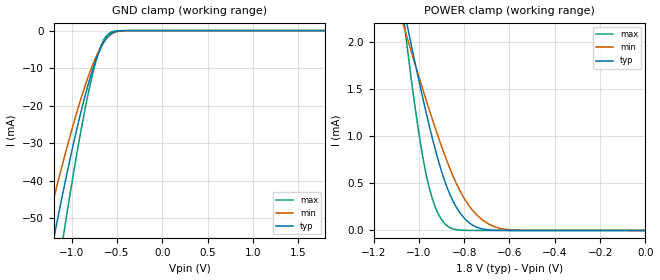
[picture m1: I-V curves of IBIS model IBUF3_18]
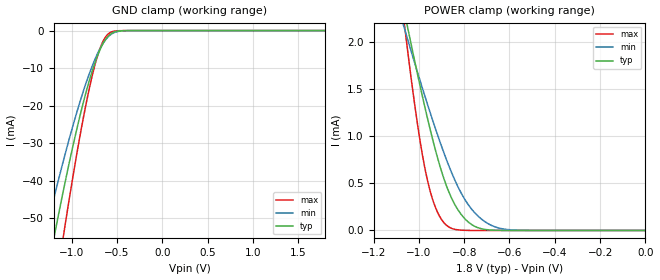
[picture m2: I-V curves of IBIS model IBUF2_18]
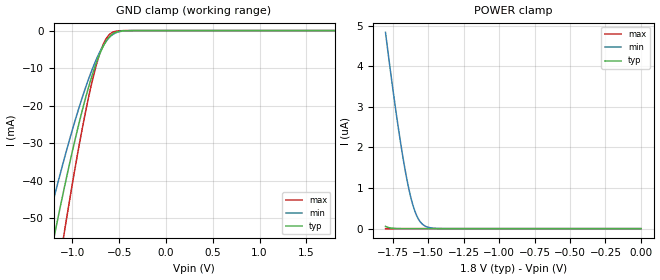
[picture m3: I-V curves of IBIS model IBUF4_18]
| TEXAS INSTRUMENTS INCORPORATED
| High Precision Analog Group
| IBIS Model of TLV320AIC3204
| Ultra Low Power Stereo Audio Codec
| part#   Digital Voltage Range   Package-type   #pin
| TLV320AIC3204RHBT   1.65V-1.95V   QFN   32
| TLV320AIC3204RHBR   1.65V-1.95V   QFN   32
[IBIS Ver]   4.0
[Comment char]  |_char
[File Name]   tlv320aic3204.ibs
[File Rev]   1.2 | E
[Date]   April 10, 2012
[Source]   Data created from TI-SPICE simulations at TI-HPA.
[Notes]   IBIS models created for IOVDD=DVDD=1.8/1.65/1.95 voltage range.
[Disclaimer] Property of Texas Instruments Incorporated.  Unauthorized
   reproduction and/or distribution is strictly prohibited.
   This product is protected under copyright law.
   Created  2012, (C) Copyright  2008, Texas Instruments
   Incorporated, All Rights Reserved
   UNLESS THERE IS A SIGNED, WRITTEN AGREEMENT TO THE
   CONTRARY, TEXAS INSTRUMENTS (TI) IS PROVIDING THE IBIS
   MODELS  AND WITHOUT ANY WARRANTY, EXPRESSED OR
   IMPLIED.  TI assumes no liability for:
   1) the accuracy of the IBIS models provided to your
   company;
   2) the proper functioning of these IBIS Models in your
   design or for any resulting applications; or
   3) infringement of patents, copyrights or intellectual
   property rights resulting from your use of these IBIS
   models.
   TI provides IBIS Models as a service to our customers.
   You and your company shall not distribute, sell or give
   these models to anyone else without prior written
   permission from TI.
   TI reserves the right to make changes to our products or
   to discontinue any semiconductor product or service
   without notice, and advises our customers to obtain the
   latest version of relevant information to verify, before
   placing orders, that the information being relied on is
   current.
   Please be aware that your receipt and use of the IBIS
   information provided shall serve as acceptance of these
   terms and conditions.  If you do not accept these terms,
   you should return or destroy the IBIS models and any
   other accompanying information immediately.
| Component TLV320AIC3204
[Component]   TLV320AIC3204
[Manufacturer]   Texas Instruments, Inc.
[Package]
|   typ   min   max
R_pkg   0.0761   0.0299   0.1101
L_pkg   1.1413nH   0.7391nH   1.5998nH
C_pkg   0.1818pF   0.1548pF   0.2745pF
[Pin]   signal_name   model_name   R_pin   L_pin   C_pin
1   MCLK   IBUF3_18   0.0843   1.21035nH   0.15565pF
2   BCLK   IOBUF_18   0.07376   1.04734nH   0.16399pF
3   WCLK   IOBUF_18   0.06637   0.94061nH   0.15628pF
4   DIN_MFP1   IBUF3_18   0.06804   0.96386nH   0.15867pF
5   DOUT_MFP2   OBUF2_18   0.07842   1.11449nH   0.17348pF
6   IOVDD   POWER   0.09718   1.3981nH   0.1889pF
7   IOVSS   GND   0.07358   1.04468nH   0.16245pF
8   SCLK_MFP3   IBUF4_18   0.08662   1.24526nH   0.15856pF
9   SCL_SSZ   I2CBUF_18   0.09486   1.37075nH   0.16588pF
10   SDA_MOSI   I2CBUF_18   0.08551   1.22071nH   0.17615pF
11   MISO_MFP4   OBUF1_18   0.08354   1.1883nH   0.1739pF
12   SPI_SELECT   IBUF1_18   0.08888   1.26731nH   0.17521pF
13   IN1_L   NC   0.10506   1.52032nH   0.19276pF
14   IN1_R   NC   0.09092   1.30262nH   0.18492pF
15   IN2_L   NC   0.0837   1.19263nH   0.17435pF
16   IN2_R   NC   0.095   1.36986nH   0.17145pF
17   AVSS   GND   0.04502   0.98171nH   0.20452pF
18   REF   NC   0.07598   1.07406nH   0.17015pF
19   MICBIAS   NC   0.08288   1.1762nH   0.17166pF
20   IN3_L   NC   0.07046   0.99184nH   0.16153pF
21   IN3_R   NC   0.06587   0.92585nH   0.15484pF
22   LOL   NC   0.06756   0.95011nH   0.15852pF
23   LOR   NC   0.0803   1.1385nH   0.17871pF
24   AVDD   POWER   0.0437   0.89119nH   0.20777pF
25   HPL   NC   0.11011   1.59985nH   0.18762pF
26   LDOIN_HPVDD   POWER   0.04871   1.0902nH   0.22686pF
27   HPR   NC   0.0491   0.74997nH   0.27451pF
28   DVSS   GND   0.04558   1.00319nH   0.21651pF
29   DVDD   POWER   0.02991   0.73918nH   0.25324pF
30   LDO_SELECT   NC   0.08352   1.18799nH   0.17586pF
31   RESETB   IBUF2_18   0.08629   1.23261nH   0.17795pF
32   GPIO_MFP5   IOBUF_18   0.09629   1.39283nH   0.16735pF
| Models and submodels in the file (8): IBUF3_18 (Input), IBUF1_18 (Input), IBUF2_18 (Input), IBUF4_18 (Input), IOBUF_18 (I/O), I2CBUF_18 (I/O_open_drain), OBUF2_18 (Output), OBUF1_18 (Output)
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[Model]   IBUF3_18
Model_type  Input
Vinl=0.495
Vinh=1.365
| variable   typ   min   max
C_comp   1.31pF   1.15pF   1.43pF
[Temperature Range]   40   100   -40
| Ambient temperature   25   85   -40
[Voltage range]   1.8   1.65   1.95
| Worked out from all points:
|   GND clamp passes 1 mA (typ) near -0.57 V on its own axis
|   POWER clamp passes 1 mA (typ) near -0.94 V on its own axis
[GND Clamp]
| IBUF3_18
|   Voltage   I(typ)   I(min)   I(max)
-1.8V     -137.6mA   -110mA     -176.5mA
-1.29V    -67.21mA   -54.1mA    -87.09mA
-1.18V    -53.33mA   -43.13mA   -68.94mA
-1.08V    -41.34mA   -33.68mA   -53.07mA
-910mV    -22.93mA   -19.14mA   -28.35mA
-785mV    -11.72mA   -10.2mA    -13.28mA
-730mV    -7.711mA   -6.953mA   -8.032mA
-675mV    -4.471mA   -4.268mA   -4.022mA
-625mV    -2.333mA   -2.42mA    -1.689mA
-575mV    -1.009mA   -1.184mA   -542.1uA
-390mV    -10.81uA   -26.47uA   -1.124uA
1.8V      39.03pA    509.5pA    14.13pA
[POWER Clamp]
| IBUF3_18
|   Voltage   I(typ)   I(min)   I(max)
-1.8V     11.83mA    8.628mA    19.35mA
-1.065V   2.333mA    2.152mA    2.209mA
-1.055V   2.216mA    2.07mA     2.012mA
-1.045V   2.1mA      1.989mA    1.819mA
-1V       1.591mA    1.63mA     1.031mA
-960mV    1.169mA    1.323mA    510.8uA
-915mV    749uA      995.8uA    180.4uA
-860mV    365.8uA    639.8uA    27.05uA
-815mV    175.7uA    404.5uA    3.749uA
-775mV    76.29uA    250.6uA    597.6nA
-655mV    1.92uA     31.22uA    2.358nA
-16.28fV  39.03pA    476.1pA    17.07pA
[Model]   IBUF2_18
Model_type  Input
Vinl=0.495
Vinh=1.365
| variable   typ   min   max
C_comp   1.31pF   1.15pF   1.42pF
[Temperature Range]   40   100   -40
| Ambient temperature   25   85   -40
[Voltage range]   1.8   1.65   1.95
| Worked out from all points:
|   GND clamp passes 1 mA (typ) near -0.57 V on its own axis
|   POWER clamp passes 1 mA (typ) near -0.94 V on its own axis
[GND Clamp]
| IBUF2_18
|   Voltage   I(typ)   I(min)   I(max)
-1.8V     -137.6mA   -110mA     -176.5mA
-1.29V    -67.21mA   -54.1mA    -87.09mA
-1.18V    -53.33mA   -43.13mA   -68.94mA
-1.08V    -41.34mA   -33.68mA   -53.07mA
-910mV    -22.93mA   -19.14mA   -28.35mA
-785mV    -11.72mA   -10.2mA    -13.28mA
-730mV    -7.711mA   -6.953mA   -8.032mA
-675mV    -4.471mA   -4.268mA   -4.022mA
-625mV    -2.333mA   -2.42mA    -1.689mA
-575mV    -1.009mA   -1.184mA   -542.1uA
-390mV    -10.81uA   -26.47uA   -1.124uA
1.8V      39.03pA    509.5pA    14.13pA
[POWER Clamp]
| IBUF2_18
|   Voltage   I(typ)   I(min)   I(max)
-1.8V     11.83mA    8.628mA    19.35mA
-1.065V   2.333mA    2.152mA    2.209mA
-1.055V   2.216mA    2.07mA     2.012mA
-1.045V   2.1mA      1.989mA    1.819mA
-1V       1.591mA    1.63mA     1.031mA
-960mV    1.169mA    1.323mA    510.8uA
-915mV    749uA      995.8uA    180.4uA
-860mV    365.8uA    639.8uA    27.05uA
-815mV    175.7uA    404.5uA    3.749uA
-775mV    76.29uA    250.6uA    597.6nA
-655mV    1.92uA     31.22uA    2.358nA
-16.28fV  39.03pA    476.1pA    17.07pA
[Model]   IBUF4_18
Model_type  Input
Vinl=0.495
Vinh=1.365
| variable   typ   min   max
C_comp   1.34pF   1.12pF   1.47pF
[Temperature Range]   40   100   -40
| Ambient temperature   25   85   -40
[Voltage range]   1.8   1.65   1.95
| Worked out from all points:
|   GND clamp passes 1 mA (typ) near -0.57 V on its own axis
[GND Clamp]
| IBUF4_18
|   Voltage   I(typ)   I(min)   I(max)
-1.8V     -137.6mA   -110mA     -176.5mA
-1.29V    -67.21mA   -54.1mA    -87.09mA
-1.18V    -53.33mA   -43.13mA   -68.94mA
-1.08V    -41.34mA   -33.68mA   -53.07mA
-910mV    -22.93mA   -19.14mA   -28.35mA
-785mV    -11.72mA   -10.2mA    -13.28mA
-730mV    -7.711mA   -6.953mA   -8.032mA
-675mV    -4.471mA   -4.268mA   -4.022mA
-625mV    -2.333mA   -2.42mA    -1.689mA
-575mV    -1.009mA   -1.184mA   -542.1uA
-390mV    -10.81uA   -26.47uA   -1.124uA
1.8V      40.23pA    492.9pA    15.03pA
[POWER Clamp]
| IBUF4_18
|   Voltage   I(typ)   I(min)   I(max)
-1.8V     57.58nA    4.834uA    44.47pA
-1.755V   11.48nA    3.619uA    43.84pA
-1.715V   2.689nA    2.614uA    43.29pA
-1.68V    790pA      1.819uA    42.81pA
-1.65V    309pA      1.228uA    42.39pA
-1.62V    150.2pA    748.7nA    41.98pA
-1.595V   102.8pA    451.6nA    41.64pA
-1.565V   81.55pA    219.9nA    41.22pA
-1.535V   74.15pA    97.12nA    40.81pA
-1.49V    70.52pA    26.03nA    40.19pA
-1.41V    68.3pA     2.775nA    39.08pA
-16.28fV  40.23pA    477.2pA    18.27pA
